FUNCTION_BLOCK FB 131
TITLE =TRASFERIMENTO PARAMETRI AZIONAMENTO 1 MASTER
VERSION : 0.1

BEGIN
NETWORK
TITLE =START SCRITTURA PARAMETRO 1 SE VIENE VARIATO PKE/INDEX/VALORE
//I07 (RISOLUZIONE)
//


      L     DB100.DBD  100;
      L     DB101.DBD  100;
      ==D   ;
      SPB   _006;

      L     1160;
      T     DB101.DBW   20;

      L     7;
      T     DB101.DBW   22;

      L     DB100.DBD  100;
      T     DB101.DBD   24;
      =     M      3.0;
_006: NOP   0;

NETWORK
TITLE =START SCRITTURA PARAMETRO 2 SE VIENE VARIATO PKE/INDEX/VALORE
//I08 NUMERO GIRI DI RISOLUZIONE
      L     DB100.DBD  104;
      L     DB101.DBD  104;
      ==D   ;
      SPB   _007;

      L     1160;
      T     DB101.DBW   20;

      L     8;
      T     DB101.DBW   22;

      L     DB100.DBD  104;
      T     DB101.DBD   24;
      =     M      3.1;
_007: NOP   0;

NETWORK
TITLE =START SCRITTURA PARAMETRO 3 SE VIENE VARIATO PKE/INDEX/VALORE
//I10 MASSIMA VELOCITA'
//
      L     DB100.DBD  108;
      L     DB101.DBD  108;
      ==D   ;
      SPB   _008;

      L     1160;
      T     DB101.DBW   20;
      L     10;
      T     DB101.DBW   22;
      L     DB100.DBD  108;
      T     DB101.DBD   24;
      =     M      3.2;

_008: NOP   0;

NETWORK
TITLE =START SCRITTURA PARAMETRO 4 SE VIENE VARIATO PKE/INDEX/VALORE
//I11 MAX ACCELERAZIONE MOTORE
      L     DB100.DBD  112;
      L     DB101.DBD  112;
      ==D   ;
      SPB   _009;

      L     1160;
      T     DB101.DBW   20;
      L     11;
      T     DB101.DBW   22;
      L     DB100.DBD  112;
      T     DB101.DBD   24;
      =     M      3.3;
_009: NOP   0;

NETWORK
TITLE =START SCRITTURA PARAMETRO 5 SE VIENE VARIATO PKE/INDEX/VALORE
//D12 VELOCITA' MANUALE
//
      L     DB100.DBD  116;
      L     DB101.DBD  116;
      ==D   ;
      SPB   _010;

      L     1560;
      T     DB101.DBW   20;
      L     12;
      T     DB101.DBW   22;
      L     DB100.DBD  116;
      T     DB101.DBD   24;
      =     M      3.4;
_010: NOP   0;

NETWORK
TITLE =START SCRITTURA PARAMETRO 6 SE VIENE VARIATO PKE/INDEX/VALORE
//I20 KP GUADAGNO
      L     DB100.DBD  120;
      L     DB101.DBD  120;
      ==D   ;
      SPB   _011;

      L     1160;
      T     DB101.DBW   20;
      L     20;
      T     DB101.DBW   22;
      L     DB100.DBD  120;
      T     DB101.DBD   24;
      =     M      3.5;
_011: NOP   0;

NETWORK
TITLE =START SCRITTURA PARAMETRO 7 SE VIENE VARIATO PKE/INDEX/VALORE
//I21 MAX ERRORE INSEGUIMENTO
//
      L     DB100.DBD  124;
      L     DB101.DBD  124;
      ==D   ;
      SPB   _012;

      L     1160;
      T     DB101.DBW   20;
      L     21;
      T     DB101.DBW   22;
      L     DB100.DBD  124;
      T     DB101.DBD   24;
      =     M      3.6;
_012: NOP   0;

NETWORK
TITLE =START SCRITTURA PARAMETRO 8 SE VIENE VARIATO PKE/INDEX/VALORE
//J10 QUOTA MISURA TAGLIO PEZZO
//
//
//
      L     DB100.DBD  128;
      L     "DatiVari".SpessoreLama;
      +D    ;
      L     DB101.DBD  128;
      ==D   ;
      SPB   _013;
      L     1180;
      T     DB101.DBW   20;
      L     10;
      T     DB101.DBW   22;
      L     DB100.DBD  128;
      L     "DatiVari".SpessoreLama;
      +D    ;
      T     DB101.DBD   24;
      =     M      3.7;
_013: NOP   0;

NETWORK
TITLE =START SCRITTURA PARAMETRO 9 SE VIENE VARIATO PKE/INDEX/VALORE
//J12 VELOCITA' DURANTE LAVORO LINEA
//
      L     DB100.DBD  132;
      L     DB101.DBD  132;
      ==D   ;
      SPB   _014;

      L     1180;
      T     DB101.DBW   20;
      L     12;
      T     DB101.DBW   22;
      L     DB100.DBD  132;
      T     DB101.DBD   24;
      =     M      4.0;
_014: NOP   0;

NETWORK
TITLE =START SCRITTURA PARAMETRO 10 SE VIENE VARIATO PKE/INDEX/VALORE
//J13 ACCELERAZIONE DURANTE LAVORO LINEA
      L     DB100.DBD  136;
      L     DB101.DBD  136;
      ==D   ;
      SPB   _015;
      L     1180;
      T     DB101.DBW   20;
      L     13;
      T     DB101.DBW   22;
      L     DB100.DBD  136;
      T     DB101.DBD   24;
      =     M      4.1;
_015: NOP   0;

NETWORK
TITLE =START SCRITTURA PARAMETRO 11 SE VIENE VARIATO PKE/INDEX/VALORE
//J14 DECELLERAZIONE LAVORO LINEA
      L     DB100.DBD  140;
      L     DB101.DBD  140;
      ==D   ;
      SPB   _016;
      L     1180;
      T     DB101.DBW   20;
      L     14;
      T     DB101.DBW   22;
      L     DB100.DBD  140;
      T     DB101.DBD   24;
      =     M      4.2;
_016: NOP   0;

NETWORK
TITLE =START SCRITTURA PARAMETRO 12 SE VIENE VARIATO PKE/INDEX/VALORE

      L     DB100.DBD  144;
      L     DB101.DBD  144;
      ==D   ;
      SPB   _017;
      L     1180;
      T     DB101.DBW   20;
      L     30;
      T     DB101.DBW   22;
      L     DB100.DBD  144;
      T     DB101.DBD   24;
//      =     M      4.3
_017: NOP   0;

NETWORK
TITLE =START SCRITTURA PARAMETRO 13 SE VIENE VARIATO PKE/INDEX/VALORE

      L     DB100.DBD  148;
      L     DB101.DBD  148;
      ==D   ;
      SPB   _018;
      L     1180;
      T     DB101.DBW   20;
      L     30;
      T     DB101.DBW   22;
      L     DB100.DBD  148;
      T     DB101.DBD   24;
//      =     M      4.4
_018: NOP   0;

NETWORK
TITLE =START SCRITTURA PARAMETRO 14 SE VIENE VARIATO PKE/INDEX/VALORE

      L     DB100.DBD  152;
      L     DB101.DBD  152;
      ==D   ;
      SPB   _019;
      L     1180;
      T     DB101.DBW   20;
      L     30;
      T     DB101.DBW   22;
      L     DB100.DBD  152;
      T     DB101.DBD   24;
//     =     M      4.5
_019: NOP   0;

NETWORK
TITLE =START SCRITTURA PARAMETRO 15 SE VIENE VARIATO PKE/INDEX/VALORE

      L     DB100.DBD  156;
      L     DB101.DBD  156;
      ==D   ;
      SPB   _020;

      L     1180;
      T     DB101.DBW   20;
      L     30;
      T     DB101.DBW   22;
      L     DB100.DBD  156;
      T     DB101.DBD   24;
//      =     M      4.6
_020: NOP   0;

NETWORK
TITLE =START SCRITTURA PARAMETRO 16 SE VIENE VARIATO PKE/INDEX/VALORE

      L     DB100.DBD  160;
      L     DB101.DBD  160;
      ==D   ;
      SPB   _021;
      L     1180;
      T     DB101.DBW   20;
      L     30;
      T     DB101.DBW   22;
      L     DB100.DBD  160;
      T     DB101.DBD   24;
//      =     M      4.7
_021: NOP   0;

NETWORK
TITLE =START SCRITTURA PARAMETRO 17 SE VIENE VARIATO PKE/INDEX/VALORE

      L     DB100.DBD  164;
      L     DB101.DBD  164;
      ==D   ;
      SPB   _022;
      L     1180;
      T     DB101.DBW   20;
      L     30;
      T     DB101.DBW   22;
      L     DB100.DBD  164;
      T     DB101.DBD   24;
//      =     M      5.0
_022: NOP   0;

NETWORK
TITLE =START SCRITTURA PARAMETRO 18 SE VIENE VARIATO PKE/INDEX/VALORE

      L     DB100.DBD  168;
      L     DB101.DBD  168;
      ==D   ;
      SPB   _023;
      L     1180;
      T     DB101.DBW   20;
      L     30;
      T     DB101.DBW   22;
      L     DB100.DBD  168;
      T     DB101.DBD   24;
//      =     M      5.1
_023: NOP   0;

NETWORK
TITLE =START SCRITTURA PARAMETRO 19 SE VIENE VARIATO PKE/INDEX/VALORE

      L     DB100.DBD  172;
      L     DB101.DBD  172;
      ==D   ;
      SPB   _024;
      L     1180;
      T     DB101.DBW   20;
      L     30;
      T     DB101.DBW   22;
      L     DB100.DBD  172;
      T     DB101.DBD   24;
//    =     M      5.2
_024: NOP   0;

NETWORK
TITLE =START SCRITTURA PARAMETRO 20 SE VIENE VARIATO PKE/INDEX/VALORE
//D22 VELOCITA' MANUALE
//
      L     DB100.DBD  180;
      L     DB101.DBD  180;
      ==D   ;
      SPB   _027;

      L     1560;
      T     DB101.DBW   20;
      L     22;
      T     DB101.DBW   22;
      L     DB100.DBD  180;
      T     DB101.DBD   24;
      =     M      2.0;
_027: NOP   0;

NETWORK
TITLE =LETTURA PARAMETRO I80 QUOTA ATTUALE MASTER IN AUTOMATICO
//I80
//
      UN    "25SA2";
      SPB   _025;

      L     1160;
      T     DB101.DBW   20;
      L     80;
      T     DB101.DBW   22;

      L     DB101.DBD   12; // LEGGO VALORE POSIZIONE ATTUALE
      T     DB101.DBD  176; // POSIZIONE ATTUALE LETTA DA ESA

      =     M      5.3;
_025: NOP   0;

      U     "25SA2";
      SPB   _026;
      L     0;
      T     DB101.DBD  176;
_026: NOP   0;

NETWORK
TITLE =START SCRITTURA PARAMETRI
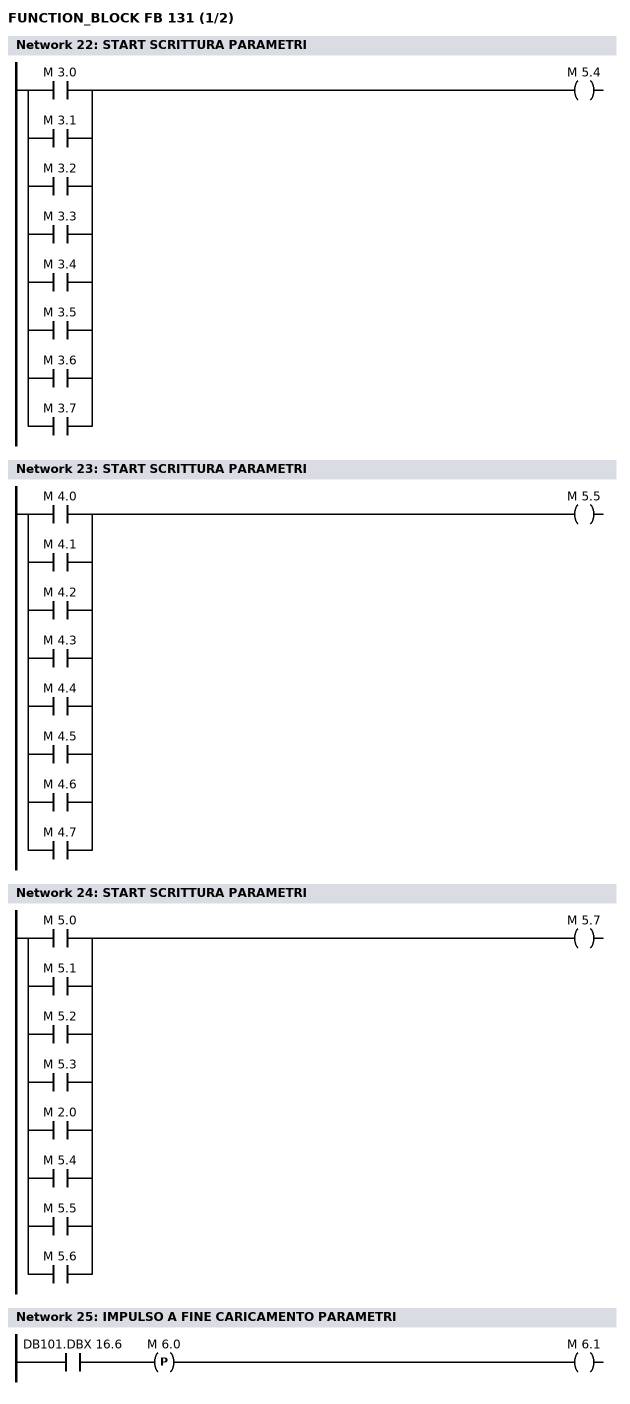
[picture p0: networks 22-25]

      O     M      3.0;
      O     M      3.1;
      O     M      3.2;
      O     M      3.3;
      O     M      3.4;
      O     M      3.5;
      O     M      3.6;
      O     M      3.7;
      =     M      5.4;
NETWORK
TITLE =START SCRITTURA PARAMETRI

      O     M      4.0;
      O     M      4.1;
      O     M      4.2;
      O     M      4.3;
      O     M      4.4;
      O     M      4.5;
      O     M      4.6;
      O     M      4.7;
      =     M      5.5;
NETWORK
TITLE =START SCRITTURA PARAMETRI

      O     M      5.0;
      O     M      5.1;
      O     M      5.2;
      O     M      5.3;
      O     M      2.0;
      O     M      5.4;
      O     M      5.5;
      O     M      5.6;
      =     M      5.7;
NETWORK
TITLE =IMPULSO A FINE CARICAMENTO PARAMETRI

      U     DB101.DBX   16.6;
      FP    M      6.0;
      =     M      6.1;
NETWORK
TITLE =START SALVATAGGIO PARAMETRI
//
//
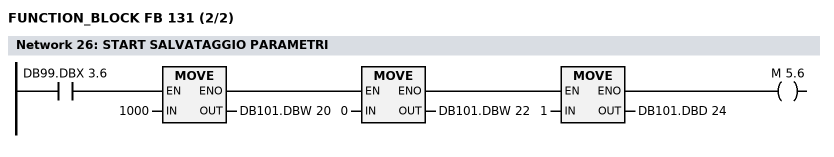
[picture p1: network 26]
      U(    ;
      U(    ;
      U     DB99.DBX    3.6;
      SPBNB _001;
      L     1000;
      T     DB101.DBW   20;
      SET   ;
      SAVE  ;
      CLR   ;
_001: U     BIE;
      )     ;
      SPBNB _002;
      L     0;
      T     DB101.DBW   22;
      SET   ;
      SAVE  ;
      CLR   ;
_002: U     BIE;
      )     ;
      SPBNB _004;
      L     1;
      T     DB101.DBD   24;
      SET   ;
      SAVE  ;
      CLR   ;
_004: U     BIE;
      =     M      5.6;
NETWORK
TITLE =VALORE DI RITORNO A COMANDO ACCETTATO

      UN    M      6.1;
      SPB   _030;
      L     DB100.DBD  100;
      T     DB101.DBD  100;
      R     M      3.0;

      L     DB100.DBD  104;
      T     DB101.DBD  104;
      R     M      3.1;

      L     DB100.DBD  108;
      T     DB101.DBD  108;
      R     M      3.2;

      L     DB100.DBD  112;
      T     DB101.DBD  112;
      R     M      3.3;

      L     DB100.DBD  116;
      T     DB101.DBD  116;
      R     M      3.4;

      L     DB100.DBD  120;
      T     DB101.DBD  120;
      R     M      3.5;

      L     DB100.DBD  124;
      T     DB101.DBD  124;
      R     M      3.6;

      L     DB100.DBD  128;
      L     "DatiVari".SpessoreLama;
      +D    ;
      T     DB101.DBD  128;
      R     M      3.7;

      L     DB100.DBD  132;
      T     DB101.DBD  132;
      R     M      4.0;

      L     DB100.DBD  136;
      T     DB101.DBD  136;
      R     M      4.1;

      L     DB100.DBD  140;
      T     DB101.DBD  140;
      R     M      4.2;

      L     DB100.DBD  144;
      T     DB101.DBD  144;
      R     M      4.3;

      L     DB100.DBD  148;
      T     DB101.DBD  148;
      R     M      4.4;

      L     DB100.DBD  152;
      T     DB101.DBD  152;
      R     M      4.5;

      L     DB100.DBD  156;
      T     DB101.DBD  156;
      R     M      4.6;

      L     DB100.DBD  160;
      T     DB101.DBD  160;
      R     M      4.7;

      L     DB100.DBD  164;
      T     DB101.DBD  164;
      R     M      5.0;

      L     DB100.DBD  168;
      T     DB101.DBD  168;
      R     M      5.1;

      L     DB100.DBD  172;
      T     DB101.DBD  172;
      R     M      5.2;

      L     DB100.DBD  176;
      T     DB101.DBD  176;
      R     M      5.3;

      L     DB100.DBD  180;
      T     DB101.DBD  180;
      R     M      2.0;
_030: NOP   0;

NETWORK
TITLE =

// AZZERAMENTO PKE QUANDO NON AVVIENE LA SCRITTURA DATI

      U     DB101.DBX   16.4; // START SCRITTURA DATI
      SPB   M001;
      L     0;
      T     DB101.DBW    8; // AZZERAMENTO PKE
      CALL "DPWR_DAT" (
           LADDR                    := W#16#100,
           RECORD                   := P#DB101.DBX 8.0 BYTE 8,
           RET_VAL                  := DB101.DBW   30);

M001: U     M      5.7;

      UN    DB101.DBX   16.4;
      S     DB101.DBX   16.4;
      R     DB101.DBX   16.5;
      R     DB101.DBX   16.6;
      UN    DB101.DBX   16.4;
      SPB   M002;

// TRASFERISCO NUMERO DEL PARAMETRO (PKE)


      L     DB101.DBW   20; // CODICE PKE
      T     DB101.DBW    8;

      U     DB101.DBX   16.4;
      R     DB101.DBX    8.3;
      S     DB101.DBX    8.4; // LANCIO JOB SCRITTURA DATI MANUALE PROF.PAG.7
//      S     DB101.DBX    8.5            // TOGLIENDO QUESTO BIT LEGGO I DATI DALLO STOBER
      R     DB101.DBX    8.6;

      U     DB101.DBX   16.4;
      UN    "25SA2";
      S     DB101.DBX    8.5; // TOGLIENDO QUESTO BIT LEGGO I DATI DALLO STOBER




// NUOVO INDEX

      L     DB101.DBW   22; // CODICE INDEX
      TAW   ;
      T     DB101.DBW   10;

// VALORE DA TRASFERIRE

      L     DB101.DBD   24; // VALORE DA TRASFERIRE
      T     DB101.DBD   12;

// LANCIO LA SCRITTURA DEI DATI

      CALL "DPWR_DAT" (
           LADDR                    := W#16#100,
           RECORD                   := P#DB101.DBX 8.0 BYTE 8,
           RET_VAL                  := DB101.DBW   32);
      SET   ;
      R     DB101.DBX   16.4;
      S     DB101.DBX   16.5; // FINE DELLA SCRITTURA DATI

// RITORNO DEI DATI TRASMESSI

      CALL "DPRD_DAT" (
           LADDR                    := W#16#100,
           RET_VAL                  := DB101.DBW   34,
           RECORD                   := P#DB101.DBX 8.0 BYTE 8);
      UN    DB101.DBX    8.4;
      U     DB101.DBX    8.5;
      UN    DB101.DBX    8.6;
      S     DB101.DBX   16.6; // DATI CORRETTAMENTE INSERITI

M002: NOP   1;

END_FUNCTION_BLOCK

